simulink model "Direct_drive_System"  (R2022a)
settings: Solver=ode5  StartTime=0.0  StopTime=T_s  FixedStep=1e-6  RelTol=1e-6
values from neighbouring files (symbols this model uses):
  bm = 3.6e-6    (= 3.6e-06)    [Direct_drive_System_mfile.m]    (also in Slider_Crank_system_mfile.m)
  D_wing = 0.5*rho*5.35e-8    (= 3.276875e-08)    [Direct_drive_System_mfile.m]    (also in Slider_Crank_system_mfile.m)
  Jm = 1.5e-7    (= 1.5e-07)    [Direct_drive_System_mfile.m]
  Jw = 7.205e-8    (= 7.205e-08)    [Direct_drive_System_mfile.m]
  Kb = 1e-2    (= 0.01)    [Direct_drive_System_mfile.m]
  Ks = (Jw+Jm)*(f0)^2    [Direct_drive_System_mfile.m]
  L = 29e-6    (= 2.9e-05)    [Direct_drive_System_mfile.m]    (also in Slider_Crank_system_mfile.m)
  L_wing = 0.5*rho*1.3045e-6    (= 7.9900625e-07)    [Direct_drive_System_mfile.m]    (also in Slider_Crank_system_mfile.m)
  Ra = 9    [Direct_drive_System_mfile.m]    (also in Slider_Crank_system_mfile.m)
  Vs = 3    [Direct_drive_System_mfile.m]
undefined symbols (not defined in the file or in its folder): f0, r

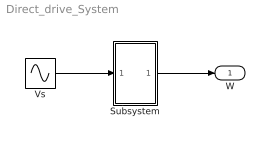
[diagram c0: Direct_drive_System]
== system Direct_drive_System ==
  Subsystem : Subsystem
  Vs : Sin  Amplitude=Vs  Frequency=f0  SampleTime=0
  W : Outport  VectorParamsAs1DForOutWhenUnconnected=off
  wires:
  Subsystem/1(W) -> W/1
  Vs/1 -> Subsystem/1(In1)

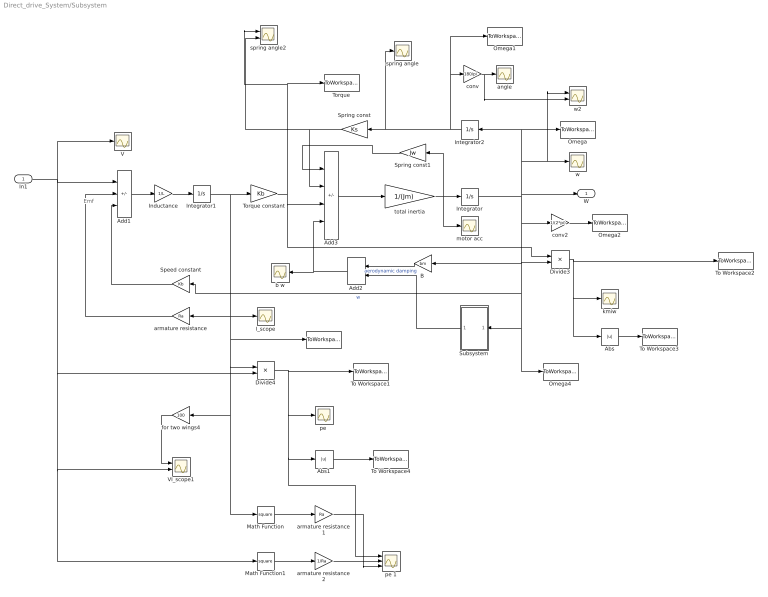
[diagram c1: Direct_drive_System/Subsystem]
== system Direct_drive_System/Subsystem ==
  note: Emf
  In1 : Inport
  Abs : Abs
  Abs1 : Abs
  Add1 : Sum  Inputs=+--
  Add2 : Sum
  Add3 : Sum  Inputs=--+-
  "B " : Gain  Gain=bm
  Divide3 : Product  Inputs=**
  Divide4 : Product  Inputs=**
  I : ToWorkspace  VariableName=I  SaveFormat=Timeseries  SampleTime=-1
  I_scope : Scope
  Inductance : Gain  Gain=1/L
  Integrator : Integrator
  Integrator1 : Integrator
  Integrator2 : Integrator
  Math Function : Math  Operator=square
  Math Function1 : Math  Operator=square
  Omega : ToWorkspace  VariableName=Omega  SaveFormat=Timeseries  SampleTime=-1
  Omega1 : ToWorkspace  VariableName=Theta  SaveFormat=Timeseries  SampleTime=-1
  Omega2 : ToWorkspace  VariableName=Frequency  SaveFormat=Timeseries  SampleTime=-1
  Omega4 : ToWorkspace  VariableName=Speed  SaveFormat=Timeseries  SampleTime=-1
  Speed constant : Gain  Gain=Kb
  Spring const : Gain  Gain=Ks
  Spring const1 : Gain  Gain=Jw
  Subsystem : Subsystem
  To Workspace1 : ToWorkspace  VariableName=Pe  SaveFormat=Timeseries  SampleTime=-1
  To Workspace2 : ToWorkspace  VariableName=Pm  SaveFormat=Timeseries  SampleTime=-1
  To Workspace3 : ToWorkspace  VariableName=KmIW_abs  SaveFormat=Timeseries  SampleTime=-1
  To Workspace4 : ToWorkspace  VariableName=Pe_abs  SaveFormat=Timeseries  SampleTime=-1
  Torque : ToWorkspace  VariableName=Torque  SaveFormat=Timeseries  SampleTime=-1
  Torque constant : Gain  Gain=Kb
  V : Scope
  VI_scope1 : Scope  NumInputPorts=2
  angle : Scope
  armature resistance : Gain  Gain=Ra
  armature resistance1 : Gain  Gain=Ra
  armature resistance2 : Gain  Gain=1/Ra
  b w : Scope
  conv : Gain  Gain=180/pi
  conv2 : Gain  Gain=1/(2*pi)
  for two wings4 : Gain  Gain=100
  kmiw : Scope
  motor acc : Scope
  "pe " : Scope
  pe 1 : Scope  NumInputPorts=3
  spring angle : Scope
  spring angle2 : Scope  NumInputPorts=2
  total inertia : Gain  Gain=1/(Jm)
  w : Scope
  w2 : Scope  NumInputPorts=2
  W : Outport  VectorParamsAs1DForOutWhenUnconnected=off
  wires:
  Torque constant/1 -> Divide3/1, Add3/3, spring angle2/1, Torque/1
  Speed constant/1 -> Add1/3
  Integrator1/1 -> I/1, Math Function/1, for two wings4/1, Divide4/1, I_scope/1, armature resistance/1, Torque constant/1
  conv2/1 -> Omega2/1
  armature resistance/1 -> Add1/2
  Add3/1 -> total inertia/1
  Integrator2/1 -> Omega1/1, conv/1, spring angle/1, Spring const/1
  Inductance/1 -> Integrator1/1
  total inertia/1 -> Spring const1/1, Integrator/1, motor acc/1
  In1/1 -> V/1, Divide4/2, VI_scope1/2, Math Function1/1, Add1/1
  Abs1/1 -> To Workspace4/1
  Add1/1 -> Inductance/1
  Integrator/1 -> W/1, w2/1, w/1, Omega/1, Integrator2/1, Omega4/1, Subsystem/1(In1), Speed constant/1, "B "/1, Divide3/2, conv2/1  "w"
  Spring const/1 -> Add3/2, spring angle2/2
  Abs/1 -> To Workspace3/1
  conv/1 -> w2/2, angle/1
  Divide4/1 -> To Workspace1/1, pe 1/1, Abs1/1, "pe "/1
  Add2/1 -> b w/1, Add3/4
  Subsystem/1(Out1) -> Add2/2  "aerodynamic damping"
  "B "/1 -> Add2/1
  armature resistance1/1 -> pe 1/3
  Math Function/1 -> armature resistance1/1
  armature resistance2/1 -> pe 1/2
  Math Function1/1 -> armature resistance2/1
  Divide3/1 -> To Workspace2/1, Abs/1, kmiw/1
  for two wings4/1 -> VI_scope1/1
  Spring const1/1 -> Add3/1

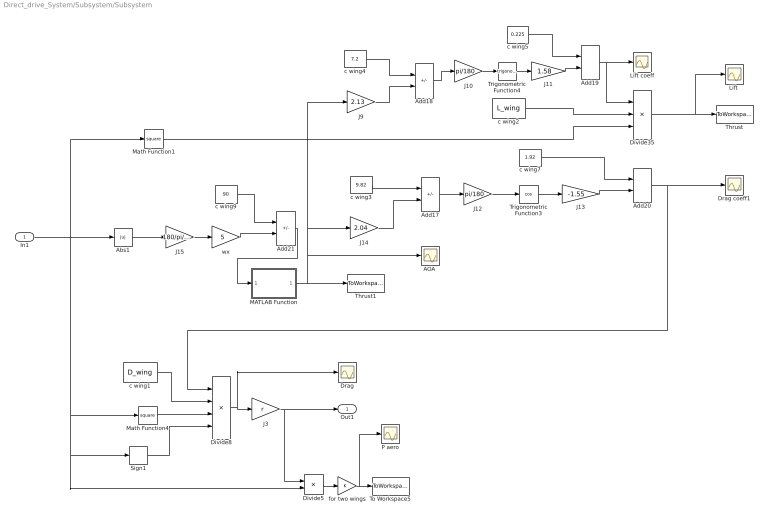
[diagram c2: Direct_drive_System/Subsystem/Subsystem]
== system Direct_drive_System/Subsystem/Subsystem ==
  In1 : Inport
  "AOA " : Scope
  Abs1 : Abs
  Add17 : Sum  Inputs=-+
  Add18 : Sum  Inputs=-+
  Add19 : Sum
  Add20 : Sum
  Add21 : Sum  Inputs=+-
  Divide35 : Product  Inputs=***
  Divide5 : Product  Inputs=**
  Divide8 : Product  Inputs=****
  Drag : Scope
  Drag coeff1 : Scope
  J10 : Gain  Gain=pi/180
  J11 : Gain  Gain=1.58
  J12 : Gain  Gain=pi/180
  J13 : Gain  Gain=-1.55
  J14 : Gain  Gain=2.04
  J15 : Gain  Gain=180/pi/1000
  J3 : Gain  Gain=r
  J9 : Gain  Gain=2.13
  "Lift " : Scope
  Lift coeff : Scope
  MATLAB Function : MATLAB Function  TreatAsAtomicUnit=on
  Math Function1 : Math  Operator=square  SignedPower=on
  Math Function4 : Math  Operator=square  SignedPower=on
  P aero : Scope
  Sign1 : Signum
  Thrust : ToWorkspace  VariableName=Lift  SaveFormat=Timeseries  SampleTime=-1
  Thrust1 : ToWorkspace  VariableName=AOA  SaveFormat=Timeseries  SampleTime=-1
  To Workspace5 : ToWorkspace  VariableName=P_aero  SaveFormat=Timeseries  SampleTime=-1
  Trigonometric Function3 : Trigonometry  Operator=cos
  Trigonometric Function4 : Trigonometry
  c wing1 : Constant  Value=D_wing
  c wing2 : Constant  Value=L_wing
  c wing3 : Constant  Value=9.82
  c wing4 : Constant  Value=7.2
  c wing5 : Constant  Value=0.225
  c wing7 : Constant  Value=1.92
  c wing9 : Constant  Value=90
  for two wings : Gain
  wx : Gain  Gain=5
  Out1 : Outport
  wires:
  Divide5/1 -> for two wings/1
  for two wings/1 -> P aero/1, To Workspace5/1
  Abs1/1 -> J15/1
  Add18/1 -> J10/1
  c wing9/1 -> Add21/1
  wx/1 -> Add21/2
  J12/1 -> Trigonometric Function3/1
  J11/1 -> Add19/2
  c wing3/1 -> Add17/1
  Trigonometric Function3/1 -> J13/1
  J13/1 -> Add20/2
  J14/1 -> Add17/2
  Add20/1 -> Divide8/1, Drag coeff1/1
  c wing5/1 -> Add19/1
  c wing4/1 -> Add18/1
  Add21/1 -> MATLAB Function/1(u)
  Add17/1 -> J12/1
  c wing2/1 -> Divide35/2
  c wing7/1 -> Add20/1
  Add19/1 -> Lift coeff/1, Divide35/1
  J10/1 -> Trigonometric Function4/1
  Divide35/1 -> Thrust/1, "Lift "/1
  Trigonometric Function4/1 -> J11/1
  J15/1 -> wx/1
  J9/1 -> Add18/2
  Math Function4/1 -> Divide8/3
  c wing1/1 -> Divide8/2
  Divide8/1 -> J3/1, Drag/1
  Sign1/1 -> Divide8/4
  MATLAB Function/1(y) -> Thrust1/1, "AOA "/1, J14/1, J9/1
  Math Function1/1 -> Divide35/3
  In1/1 -> Math Function1/1, Math Function4/1, Divide5/2, Sign1/1, Abs1/1
  J3/1 -> Out1/1, Divide5/1

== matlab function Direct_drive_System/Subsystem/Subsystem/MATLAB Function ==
function y = fcn(u)

if u >= 45
    y = u;
elseif u <= -45
    y = u;
else 
    y= 45;
end
